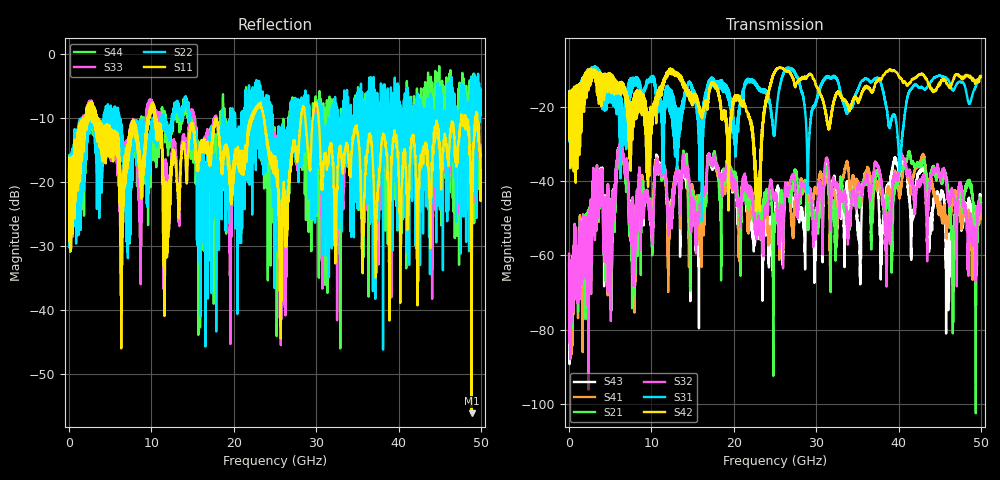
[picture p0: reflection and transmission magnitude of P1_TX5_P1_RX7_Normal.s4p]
!Keysight Technologies,N5225B,MY57041031,A.13.20.10
!Date: Friday, May 31, 2019 11:24:20
!Correction: S11(Full 4 Port(1,2,3,4))
!S12(Full 4 Port(1,2,3,4))
!S13(Full 4 Port(1,2,3,4))
!S14(Full 4 Port(1,2,3,4))
!S21(Full 4 Port(1,2,3,4))
!S22(Full 4 Port(1,2,3,4))
!S23(Full 4 Port(1,2,3,4))
!S24(Full 4 Port(1,2,3,4))
!S31(Full 4 Port(1,2,3,4))
!S32(Full 4 Port(1,2,3,4))
!S33(Full 4 Port(1,2,3,4))
!S34(Full 4 Port(1,2,3,4))
!S41(Full 4 Port(1,2,3,4))
!S42(Full 4 Port(1,2,3,4))
!S43(Full 4 Port(1,2,3,4))
!S44(Full 4 Port(1,2,3,4))
!S4P File: Measurements: <S11,S12,S13,S14>,
!<S21,S22,S23,S24>,
!<S31,S32,S33,S34>,
!<S41,S42,S43,S44>:
# Hz S  dB  R 50.0
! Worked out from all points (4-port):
!   5000 points, 10 MHz to 50 GHz, reference 50 ohm
!   strongest paths, dB at 10 MHz, 12.51 GHz, 25.01 GHz, 37.51 GHz, 50 GHz:
!     S42: -19.7, -10.0, -10.7, -12.8, -12.0
!     S31: -19.3, -23.0, -26.1, -12.3, -11.7
!     S32: -59.6, -45.9, -44.6, -35.9, -47.2
!     S21: -65.0, -46.3, -49.0, -37.8, -47.1
!     S41: -62.5, -44.5, -48.6, -40.6, -46.9
!     S43: -62.0, -43.9, -46.8, -42.4, -45.9
!   lowest |S11| = -56.1 dB at 48.87 GHz (marker M1), VSWR 1.00, Z = 50.1 - j0.126 ohm
!   |S11| at or under -10 dB: 3.502 GHz to 9.556 GHz (6.054 GHz wide, 92.7 % of centre); 10.5 GHz to 22.11 GHz (11.6 GHz wide, 71.2 % of centre); 30.29 GHz to 47.6 GHz (17.3 GHz wide, 44.4 % of centre)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
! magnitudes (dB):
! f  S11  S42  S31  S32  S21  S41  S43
! 10 MHz  -19.7  -19.7  -19.3  -59.6  -65.0  -62.5  -62.0
! 6.21 GHz  -18.7  -16.5  -17.5  -29.3  -29.6  -30.0  -29.7
! 7.86 GHz  -11.4  -21.1  -12.4  -57.8  -58.4  -57.9  -57.0
! 22.93 GHz  -8.3  -39.7  -14.7  -53.3  -47.0  -45.8  -49.4
! 25.42 GHz  -21.1  -9.6  -16.5  -54.0  -54.8  -54.0  -43.4
! 48.87 GHz  -56.1  -12.1  -17.6  -51.5  -42.8  -53.6  -50.7
! 50 GHz  -18.2  -12.0  -11.7  -47.2  -47.1  -46.9  -45.9
